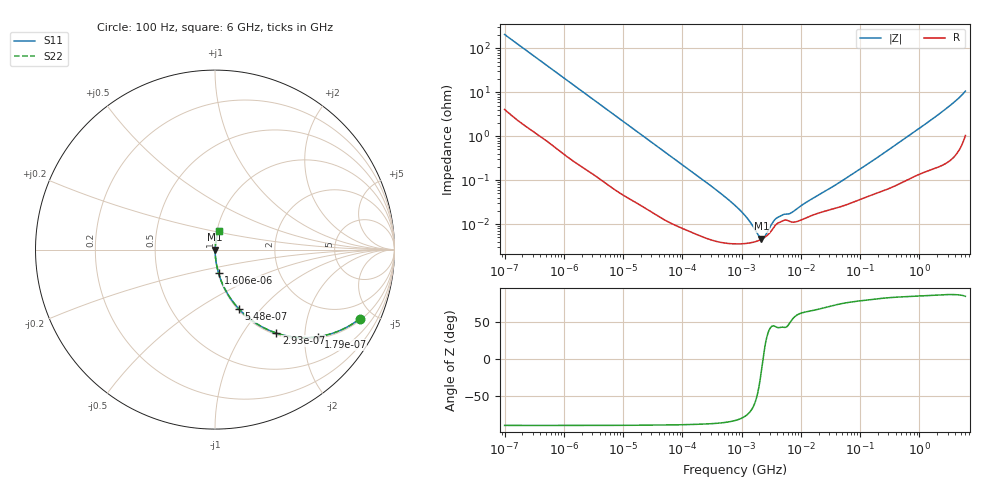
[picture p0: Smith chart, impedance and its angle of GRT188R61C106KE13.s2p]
!Murata Part Number: GRT188R61C106KE13
!These Parameters are Measured in Series Mode Connection
!Data Generated on Jun 19, 2026
!  o--ll--o
!Port1  Port2
!  o------o
!Operation Temp=25[degC], DC Bias Voltage=0[V]
!Freq. Start=100[Hz] Stop=6[GHz] 401[Steps]
# Hz S RI R 50
!Freq.(Hz) S11(Real) S11(Imag) S21(Real) S21(Imag) S12(Real) S12(Imag) S22(Real) S22(Imag)
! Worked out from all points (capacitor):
!   401 points, 100 Hz to 6 GHz, reference 50 ohm
!   read as one part in series: C = 7.65 uF near 109 Hz
!   lowest |Z| = 4.67 mohm at 2.169 MHz (marker M1)
!   series resonance near 2.298 MHz, so ESL is about 630 pH
!   S11 on the Smith chart (normalised r, x): 100 Hz: 1.08, -4.14; 179 Hz: 1.04, -2.33; 293 Hz: 1.03, -1.43; 548 Hz: 1.01, -0.77; 1.606 kHz: 1.00, -0.27; 6 GHz: 1.02, +0.21
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100  0.8062 -0.3855  0.1938 0.3855  0.1938 0.3855  0.8062 -0.3855
179  0.5743 -0.4854  0.4257 0.4854  0.4257 0.4854  0.5743 -0.4854
293  0.3414 -0.465  0.6586 0.465  0.6586 0.465  0.3414 -0.465
548  0.1339 -0.3312  0.8661 0.3312  0.8661 0.3312  0.1339 -0.3312
897  0.0568 -0.2224  0.9432 0.2224  0.9432 0.2224  0.0568 -0.2224
1606  0.0197 -0.1302  0.9803 0.1302  0.9803 0.1302  0.0197 -0.1302
2008  0.0132 -0.1051  0.9868 0.1051  0.9868 0.1051  0.0132 -0.1051
6433  0.00181 -0.0337  0.9982 0.0337  0.9982 0.0337  0.00181 -0.0337
40335  0.000178 -0.00552  0.9998 0.00552  0.9998 0.00552  0.000178 -0.00552
316350  4.36e-05 -0.000712  1 0.000712  1 0.000712  4.36e-05 -0.000712
774597  3.55e-05 -0.000265  1 0.000265  1 0.000265  3.55e-05 -0.000265
1449809  3.78e-05 -9.67e-05  1 9.67e-05  1 9.67e-05  3.78e-05 -9.67e-05
1585629  3.88e-05 -7.71e-05  1 7.71e-05  1 7.71e-05  3.88e-05 -7.71e-05
2169299  4.52e-05 -1.18e-05  1 1.18e-05  1 1.18e-05  4.52e-05 -1.18e-05
3103719  6.74e-05 6.22e-05  0.9999 -6.22e-05  0.9999 -6.22e-05  6.74e-05 6.22e-05
4060267  0.000105 9.58e-05  0.9999 -9.58e-05  0.9999 -9.58e-05  0.000105 9.58e-05
6948629  0.000112 0.000143  0.9999 -0.000143  0.9999 -0.000143  0.000112 0.000143
1.555665e7  0.000159 0.000344  0.9998 -0.000344  0.9998 -0.000344  0.000159 0.000344
4.764863e7  0.000251 0.0009  0.9997 -0.0009  0.9997 -0.0009  0.000251 0.0009
3.124326e8  0.000675 0.00501  0.9993 -0.00501  0.9993 -0.00501  0.000675 0.00501
2.240541e9  0.00316 0.033  0.9968 -0.033  0.9968 -0.033  0.00316 0.033
6e9  0.0211 0.1028  0.9789 -0.1028  0.9789 -0.1028  0.0211 0.1028
